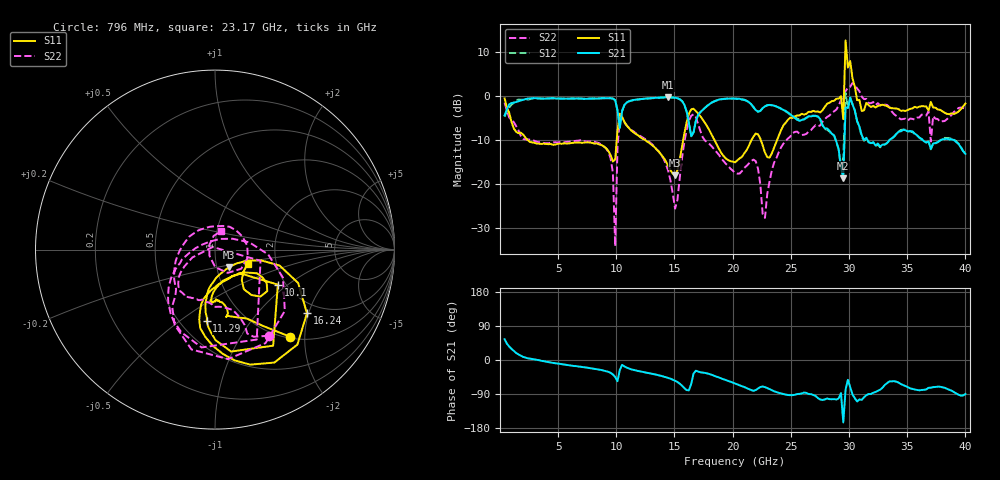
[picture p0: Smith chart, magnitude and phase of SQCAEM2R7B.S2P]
! Network Analyzer HP8722ES.07.66: Jul 25, 2000 Serial No. US39175408
! 26 Oct 2004  13:29:14
! Frequency  S11  S21  S12  S22
# HZ  S  DB R  50
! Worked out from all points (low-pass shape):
!   201 points, 400 MHz to 40 GHz, reference 50 ohm
!   highest |S21| = -0.35 dB at 14.46 GHz (marker M1); lowest = -18.7 dB at 29.51 GHz (marker M2)
!   |S21| within 3 dB of the highest: 559 MHz to 10.11 GHz (9.547 GHz wide, 179 % of centre); 10.52 GHz to 16.02 GHz (5.496 GHz wide, 41.4 % of centre)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
!   lowest |S11| = -18.1 dB at 15.05 GHz (marker M3), VSWR 1.28, Z = 57 - j11.4 ohm
!   |S11| at or under -10 dB: 2.357 GHz to 10.04 GHz (7.682 GHz wide, 124 % of centre); 12.45 GHz to 15.75 GHz (3.301 GHz wide, 23.4 % of centre); 18.41 GHz to 21.63 GHz (3.223 GHz wide, 16.1 % of centre)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
!   |S22| runs from -34.1 to 2.9 dB; largest |S21 - S12| = 0.47
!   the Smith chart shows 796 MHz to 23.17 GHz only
!   S11 on the Smith chart (normalised r, x): 796 MHz: 1.03, -1.69; 10.1 GHz: 1.82, -0.85; 11.29 GHz: 0.67, -0.64; 16.24 GHz: 1.68, -1.95; 23.17 GHz: 1.42, -0.24
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4e8  -0.60 -36.4  -4.44 54.9  -4.81 60.3  -1.57 -28.3
7.96e8  -3.88 -49.3  -1.95 35.5  -2.72 35.2  -4.95 -58.1
7.132e9  -10.69 -93.3  -0.69 -18.8  -0.69 -18.8  -10.31 -123.7
9.904e9  -14.45 -43.8  -1.02 -45.0  -1.05 -45.7  -34.15 132.4
1.0102e10  -7.94 -29.1  -3.27 -56.0  -3.43 -56.7  -11.66 -13.8
1.129e10  -7.95 -96.6  -1.12 -24.7  -1.12 -24.8  -7.80 -128.9
1.3666e10  -12.70 -99.4  -0.47 -40.6  -0.46 -40.6  -12.77 -156.1
1.4458e10  -15.99 -88.0  -0.35 -47.1  -0.40 -47.3  -17.05 -173.6
1.5052e10  -18.09 -52.2  -0.48 -54.9  -0.48 -55.1  -25.63 119.6
1.624e10  -4.10 -34.7  -6.19 -80.0  -6.25 -80.0  -5.72 -41.3
2.02e10  -15.13 -57.0  -0.70 -62.1  -0.65 -61.8  -17.53 117.1
2.317e10  -14.05 -23.9  -2.09 -77.0  -2.11 -76.9  -19.46 72.7
2.6932e10  -3.44 -32.9  -4.56 -92.4  -4.59 -92.8  -7.21 1.6
2.9506e10  -5.32 26.8  -18.71 -164.7  -13.95 -132.5  0.07 31.6
2.9704e10  12.53 -61.8  -2.67 -77.9  0.58 -56.5  1.04 -67.3
2.9902e10  6.39 -52.3  -2.76 -52.3  -2.79 -52.4  1.83 -14.4
3.0496e10  2.06 -70.8  -3.33 -100.9  -3.37 -99.0  2.50 -55.7
3.0694e10  -1.01 111.0  -5.74 -109.5  -5.82 -107.7  1.62 116.9
3.1288e10  -3.32 133.4  -10.07 -98.5  -10.24 -99.0  -0.79 112.1
3.1486e10  -1.64 -45.5  -9.53 -92.9  -9.66 -93.4  -0.73 -69.8
3.3466e10  -2.69 -36.8  -10.08 -56.5  -10.19 -56.0  -2.56 -75.4
4e10  -1.78 -50.4  -13.20 -89.8  -13.29 -90.2  -2.92 -47.1
